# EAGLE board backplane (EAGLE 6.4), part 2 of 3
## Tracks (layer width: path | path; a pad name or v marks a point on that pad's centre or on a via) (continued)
HUB_!PWRON4  (via drill 0.6) (continued)
  Top 0.254: U1.23 113.83,195.54 113.03,196.34 97.79,196.34 97.28,195.83 21.34,195.83 v20.57,196.6 | S11.1 49.42,95.36 49.02,95.76 49.02,96.77 46.48,99.31 | v11.81,98.3 12.32,97.79 25.91,97.79 28.96,100.84 44.96,100.84 46.23,99.57 46.48,99.31 | v5.59,98.42 5.33,98.55 4.32,99.57 4.32,159 20.57,175.26 v20.57,188.85 | TP38.TESTPOINT 46.48,99.31
  Bottom 0.254: v20.57,196.6 v20.57,188.85 | v11.81,98.3 5.84,98.3 v5.59,98.42
HUB_!PWRON6  (via drill 0.6)
  Top 0.254: S12.1 153.3,67.17 v153.8,66.67 | U1.32 108.45,189.75 107.7,190.5 103.63,190.5 97.28,184.15 97.28,166.12 99.57,163.83 v99.57,161.42 | v99.57,157.1 100.08,156.59 100.08,100.08 100.84,99.31 103.76,99.31 v104.01,99.06 | v106.3,99.06 106.55,99.31 122.17,99.31 v122.56,98.93 | v126.11,98.93 v128.4,98.93 | v131.19,98.93 v134.75,98.93 | v137.54,98.93 138.3,98.93 140.97,96.27 140.97,90.68 v140.59,90.3 | v140.59,88.01 140.59,86.23 149.99,76.83 v149.99,74.93
  Bottom 0.254: v153.8,66.67 152.78,67.69 152.78,69.47 151.76,70.48 151.76,74.04 150.88,74.93 v149.99,74.93 | v99.57,161.42 v99.57,157.1 | v104.01,99.06 v106.3,99.06 | v122.56,98.93 v126.11,98.93 | v128.4,98.93 v131.19,98.93 | v134.75,98.93 v137.54,98.93 138.18,98.93 139.19,99.95 TP40.TESTPOINT | v140.59,90.3 v140.59,88.01
HUB_!PWRON7  (via drill 0.6)
  Top 0.254: S10.1 148.07,157.62 v146.18,159.51 | U1.36 111.04,187.75 110.74,187.45 110.74,186.69 103.38,179.32 103.38,173.23 111.76,165.1 117.35,165.1 | 117.35,165.1 118.36,165.1 | 118.36,165.1 123.19,165.1 v123.44,164.85 | v125.73,164.85 126.11,165.23 128.02,165.23 v128.4,164.85 | v130.68,164.85 130.94,165.1 134.49,165.1 v134.75,164.85 | v137.54,164.85 138.68,164.85 142.88,160.66 v142.88,160.15 | TP42.TESTPOINT 117.86,164.59 | 117.86,164.59 117.35,165.1 | 117.86,164.59 118.36,165.1
  Bottom 0.254: v123.44,164.85 v125.73,164.85 | v128.4,164.85 v130.68,164.85 | v134.75,164.85 v137.54,164.85 | v142.88,160.15 145.54,160.15 v146.18,159.51
HUB_CFG  (via drill 0.6)
  Top 0.254: U1.40 114.81,186.22 114.81,187.71 116.46,189.36 v116.84,189.36 | v123.32,183.39 123.44,183.51 126.36,183.51 127.51,184.66 TP28.TESTPOINT
  Bottom 0.254: v116.84,189.36 117.22,188.98 117.86,188.98 118.62,188.21 118.62,186.94 122.43,183.13 123.06,183.13 v123.32,183.39
HUB_DM1
  Top 0.254: R4.1 119.45,204.47 C6.1 119.45,203.28 119.13,202.95 119.13,197.89 arc-11 119,196.34 arc14 U1.13
HUB_DM2
  Top 0.254: U1.17 116.83,198.64 113.54,201.93 113.54,202.95 113.87,203.28 C4.1 113.79,203.78 R2.1
HUB_DM3
  Top 0.254: U1.21 114.83,196.07 108.03,202.87 C8.1 108.03,204.47 R6.1
HUB_DM4
  Top 0.254: U1.26 111.12,192.75 arc-9 109.75,192.86 arc8 108.38,192.99 C12.1 107.04,192.99 R10.1
HUB_DM6
  Top 0.254: U1.34 110.26,188.75 109.22,187.71 106.5,187.71 C14.1 105.66,187.78 R12.1
HUB_DM7
  Top 0.254: U1.38 113.83,185.46 106.61,178.23 C10.1 106.61,176.53 R8.1
HUB_DP1
  Top 0.254: R3.1 118.29,204.47 C5.1 118.29,203.28 118.62,202.95 118.62,197.89 arc-9 118.49,196.34 arc9 U1.14 118.34,194.81
HUB_DP2
  Top 0.254: U1.18 116.33,198.38 113.03,201.68 113.03,202.95 112.7,203.28 C3.1 112.78,203.78 R1.1
HUB_DP3
  Top 0.254: U1.22 114.33,195.81 106.86,203.28 C7.1 106.86,204.47 R5.1
HUB_DP4
  Top 0.254: U1.27 111.12,192.25 arc2 109.73,192.23 arc-2 108.41,192.2 C11.1 107.04,192.2 R9.1
HUB_DP6
  Top 0.254: U1.35 110.53,188.25 109.22,186.94 106.5,186.94 C13.1 106.35,186.94 R11.1
HUB_DP7
  Top 0.254: U1.39 114.33,185.19 107.52,178.38 C9.1 107.52,176.53 R7.1
HUB_PORTDIS  (via drill 0.6)
  Top 0.254: U1.42 115.83,186.69 v116.59,187.45 | v125.09,181.74 126.36,181.74 127,181.1 128.02,181.1 129.29,182.37 TP30.TESTPOINT
  Bottom 0.254: v116.59,187.45 122.05,181.74 v125.09,181.74
HUB_PORTPWR  (via drill 0.6)
  Top 0.254: U1.41 115.33,187.46 116.33,188.47 117.09,188.47 v117.73,187.96 | v124.21,182.63 127.25,182.63 TP29.TESTPOINT
  Bottom 0.254: v117.73,187.96 117.73,187.07 122.17,182.37 123.95,182.37 v124.21,182.63
MOD0_5V
  Top 0.254: 107.19,321.31 107.44,321.56 | S1.1 107.69,320.81 107.19,321.31 | C33.1 106.68,320.8 107.19,321.31
  Top 1.27: J0.2 58.67,357.63 95,357.63 107.44,345.44 107.44,321.56
MOD0_5V_METERED  (via drill 1.2)
  Top 0.254: 107.19,317.76 106.93,317.5 C88.1 | S13.3 96.59,312.12 96.52,312.05 96.34,312.24 | S13.2 95.94,312.63 96.34,312.24 | C76.1 96.01,311.91 96.34,312.24 | S1.3 107.19,317.5 106.93,317.25
  Top 1.27: v45.47,186.18 39.37,192.28 17.02,192.28 8.38,200.91 8.38,274.32 23.88,289.56 84.84,289.56 v91.95,296.67 | 96.52,306.32 96.52,312.05 | 96.52,306.32 106.93,316.74 106.93,317.25 106.93,317.5 | v91.95,301.75 96.52,306.32
  Bottom 0.508: v45.47,186.18 53.59,194.06 TP16.TESTPOINT
  Bottom 1.27: J4.7 50.01,181.63 v45.47,186.18 | v91.95,296.67 v91.95,301.75
MOD0_D+_HUB-SW
  Top 0.254: R1.2 112.78,205.99 113.03,206.25 113.03,357.38 114.55,358.9 114.55,360.17 113.75,360.98 D1.4 111.8,360.98 111.63,360.81 109.98,360.81 | 109.98,360.81 109.35,360.81 108.86,361.3 U20.3 | R50.2 110.49,360.3 109.98,360.81
MOD0_D-_HUB-SW
  Top 0.254: U20.5 108.86,362.1 109.35,362.58 110.24,362.58 | R2.2 113.79,205.99 113.54,206.25 113.54,357.12 115.06,358.65 115.06,361.19 113.97,362.27 D1.2 111.94,362.27 111.63,362.58 110.24,362.58 | R51.2 110.49,362.84 110.24,362.58
MOD0_IN
  Top 0.254: J0.10 69.59,336.55 U8.7
MOD0_ISO_I2C  (via drill 0.6)
  Top 0.254: U2.5 96.27,352.04 | 96.27,352.04 R63.2 | 96.27,352.04 99.31,352.04 106.43,344.93 106.43,322.71 v106.05,322.33 | v109.35,322.33 109.35,321.18 110.49,320.04 110.49,312.17 v109.98,311.66 | v107.7,311.66 107.7,305.31 106.93,304.55 U26.11 106.93,299.72 106.43,299.21 76.2,299.21 73.91,301.5 73.91,309.37 | 73.91,309.37 73.91,309.63 74.93,310.64 R1002.2 | TP1002.TESTPOINT 88.65,309.63 74.17,309.63 73.91,309.37
  Bottom 0.254: v106.05,322.33 v109.35,322.33 | v109.98,311.66 v107.7,311.66
MOD0_ISO_POWER
  Top 0.254: S1.4 107.69,318.27 107.95,318.01 107.95,316.48 109.11,315.33 R62.2 109.11,312.94 108.58,312.42 108.58,311.02 108.2,310.64 U26.10 108.2,299.97 106.93,298.7 75.95,298.7 73.41,301.24 73.41,313.44 73.66,313.69 | 73.66,313.69 74.68,314.71 R1001.2 | TP1001.TESTPOINT 88.65,313.69 73.66,313.69
MOD0_ISO_USB  (via drill 0.6)
  Top 0.203: U20.8 106.03,362.1 105.92,362.2 v105.92,362.97
  Top 0.254: v105.92,357.63 105.92,348.49 108.46,345.95 108.46,321.31 109.98,319.79 109.98,312.93 109.09,312.04 v109.09,310.13 | 102.11,304.29 102.73,304.91 S7.6 103.74,304.91 104.14,305.31 104.14,308.36 105.92,310.13 v106.81,310.13 | 102.11,304.29 R64.2 | 102.11,304.29 102.87,303.53 104.65,303.53 105.66,302.51 U26.12 105.66,300.23 105.16,299.72 76.45,299.72 74.42,301.75 74.42,305.31 | 74.42,305.31 74.42,306.07 74.93,306.58 R1003.2 | TP1003.TESTPOINT 88.65,305.56 74.68,305.56 74.42,305.31
  Bottom 0.254: v105.92,362.97 v105.92,357.63 | v109.09,310.13 v106.81,310.13
MOD0_OUT
  Top 0.254: J0.8 46.23,362.46 46.23,361.44 64.26,343.41 U14.7
MOD0_PPS
  Top 0.254: J0.7 44.96,363.78 44.96,361.95 69.85,337.05 U8.6
MOD0_SCL
  Top 0.203: 95.11,350.92 95.36,350.67 U2.6
  Top 0.254: J0.5 48.79,365.02 50.04,363.78 50.04,359.16 58.42,350.77 91.55,350.77 R34.2 95.11,350.92
MOD0_SDA
  Top 0.203: R33.2 95.14,350.15 95.25,350.27 U2.7
  Top 0.254: J0.6 48.77,362.46 48.77,359.66 58.15,350.28 93.73,350.27 93.84,350.15 R33.2
MOD0_USB+
  Top 0.254: J0.11 41.12,365.99 43.94,368.81 74.17,368.81 81.79,361.44 100.08,361.44 102.87,358.65 105.66,358.65 107.24,360.23 U20.1
MOD0_USB-
  Top 0.254: J0.12 39.88,363.73 39.88,365.51 43.69,369.32 74.42,369.32 82.04,361.95 100.08,361.95 103.12,365 105.66,365 107.24,363.42 U20.7
MOD0_USB_!EN  (via drill 0.6)
  Top 0.254: S13.4 97.24,312.97 v99.19,311.02 | S7.4 102.73,306.21 102.36,306.58 102.36,307.85 v101.22,308.99
  Bottom 0.254: v99.19,311.02 v101.22,308.99
MOD0_USB_VBUS
  Top 0.254: C77.1 91.95,325.88 93.22,324.61 | S13.7 95.94,319.71 96.14,319.91 | 96.14,319.91 96.27,320.04 | S13.6 96.59,319.46 96.14,319.91
  Top 0.762: C95.1 95.25,322.58
  Top 1.27: J0.13 38.58,364.97 36.83,363.22 36.83,361.7 73.66,324.87 92.99,324.87 92.99,324.84 93.22,324.61 95.25,322.58 96.27,321.56 96.27,320.04
MOD0_VCCIO  (via drill 1.2)
  Top 0.203: U2.8 95.36,349.87 95.25,349.76 95.25,349.25
  Top 0.254: v89.66,349 91.19,349 91.69,349.5 R34.1 92.46,348.85 R33.1 94.85,348.85 95.25,349.25 96.01,348.49 C22.1 | C52.1 94.74,342.65 | 94.74,342.65 94.74,342.89 U14.8 | C40.1 94.74,335.79 | 94.74,335.79 94.74,336.03 U8.8 | v89.66,335.28 94.23,335.28 94.74,335.79 | v89.66,342.14 94.23,342.14 94.74,342.65
  Top 1.27: J0.4 51.28,359.44 58.67,352.04 v89.66,352.04 | v89.66,349 v89.66,345.19 | v89.66,342.14 v89.66,338.84
  Bottom 1.27: v89.66,352.04 v89.66,349 | v89.66,345.19 v89.66,342.14 | v89.66,338.84 v89.66,335.28
MOD1_5V
  Top 0.254: C34.1 163.43,332.49 163.43,331.72 163.18,331.47 S2.1
  Top 1.27: J1.2 215.42,360.2 187.2,331.72 163.43,331.72
MOD1_5V_METERED  (via drill 1.2)
  Top 0.254: S14.2 149.31,357.7 C78.1 149.53,357.05 S14.3 | 155.82,331.72 156.18,331.36 C89.1 157.33,331.97 S2.3
  Top 1.27: v145.29,363.22 145.29,358.9 | 145.29,358.9 146.81,357.38 148.99,357.38 C78.1 | 145.29,358.9 145.29,339.09 152.66,331.72 155.82,331.72 | v28.7,190.25 16.51,190.25 6.6,200.15 6.6,274.83 12.45,280.67 12.45,294.39 6.6,300.23 6.6,340.87 39.88,374.14 77.72,374.14 83.57,368.3 96.77,368.3 102.87,374.4 137.16,374.4 v145.29,366.27
  Bottom 0.508: 30.48,188.47 30.73,188.47 33.02,190.75 49.02,190.75 53.59,195.33 59.69,195.33 TP17.TESTPOINT
  Bottom 1.27: J4.8 50.01,168.63 46.48,165.1 32.51,165.35 30.48,167.39 30.48,188.47 v28.7,190.25 | v145.29,366.27 v145.29,363.22
MOD1_D+_HUB-SW
  Top 0.203: U21.3 122.79,362.6
  Top 0.254: 122.79,362.6 122.17,363.22 120.9,363.22 | R3.2 118.36,205.99 118.62,206.25 118.62,356.62 116.84,358.39 116.84,361.7 118.07,362.93 D1.8 120.1,362.93 120.4,363.22 120.9,363.22 | R52.2 121.41,363.73 120.9,363.22
MOD1_D-_HUB-SW
  Top 0.203: U21.5 122.79,361.8
  Top 0.254: R4.2 119.38,205.99 119.13,206.25 119.13,356.87 117.35,358.65 117.35,360.93 118.04,361.62 D1.6 119.96,361.62 120.27,361.31 120.9,361.31 | 120.9,361.31 122.3,361.31 122.79,361.8 | R53.2 121.41,360.81 120.9,361.31
MOD1_IN
  Top 0.254: J1.10 205.26,360.96 195.83,351.53 U9.7
MOD1_ISO_I2C  (via drill 0.6)
  Top 0.254: U3.5 R66.2 158.13,336.95 157.73,336.55 157.23,336.55 155.45,334.77 v155.45,333.25 | v158.24,323.34 U27.11 v158.24,319.28 | v158.24,325.88 158.24,326.39 v155.45,329.18 | LED1005.A TP1005.TESTPOINT 161.29,310.64 158.24,313.69 v158.24,314.71
  Bottom 0.254: v155.45,329.18 v155.45,333.25 | v158.24,323.34 v158.24,325.88 | v158.24,314.71 v158.24,319.28
MOD1_ISO_POWER  (via drill 0.6)
  Top 0.254: v159.51,323.34 U27.10 v159.51,319.28 | S2.4 158.5,331.47 158.24,331.22 158.24,329.44 158.61,329.07 | R65.2 158.61,329.07 | LED1004.A TP1004.TESTPOINT v159.51,314.71 | v159.51,325.88 159.51,328.17 158.61,329.07
  Bottom 0.254: v159.51,323.34 v159.51,325.88 | v159.51,314.71 v159.51,319.28
MOD1_ISO_USB  (via drill 0.6)
  Top 0.203: U21.8 126.13,361.8 126.24,361.7 126.26,361.42
  Top 0.254: v156.97,323.34 U27.12 v156.97,319.28 | v156.97,325.88 144.27,338.58 144.27,350.5 v143.89,350.89 143.89,350.9 142.88,351.92 130.44,351.9 126.49,355.85 126.49,356.25 R67.2 126.49,356.98 v126.49,358.52 | 126.26,361.42 126.26,360.66 v126.49,360.43 | S8.6 148.48,349.87 147.46,350.89 v146.69,350.89 | LED1006.A TP1006.TESTPOINT 162.56,306.58 156.97,312.17 v156.97,314.71
  Bottom 0.254: v143.89,350.89 v146.69,350.89 | v156.97,323.34 v156.97,325.88 | v126.49,360.43 v126.49,358.52 | v156.97,314.71 v156.97,319.28
MOD1_OUT
  Top 0.254: J1.8 207.77,362.46 207.77,360.93 192.53,345.69 U15.7
MOD1_PPS
  Top 0.254: J1.7 206.5,363.73 206.5,361.44 196.09,351.03 U9.6
MOD1_SCL
  Top 0.203: U3.6 159.91,338.18 160.13,337.96 163.29,337.96
  Top 0.254: J1.5 210.34,364.97 211.58,363.73 211.58,361.95 187.56,337.93 R36.2 163.32,337.93 163.29,337.96
MOD1_SDA
  Top 0.203: U3.7 161.02,338.58
  Top 0.254: J1.6 210.34,361.47 187.45,338.58 161.02,338.58 161.04,338.57 R35.2
MOD1_USB+
  Top 0.254: J1.11 202.72,365.74 199.39,369.06 182.63,369.06 178.56,365 126.24,365 124.91,363.67 U21.1
MOD1_USB-
  Top 0.254: J1.12 202.67,362.48 201.42,363.73 201.42,366.27 199.14,368.55 182.88,368.55 178.82,364.49 132.84,364.49 128.27,359.41 126.24,359.41 124.91,360.73 U21.7
MOD1_USB_!EN  (via drill 0.6)
  Top 0.254: S8.4 148.7,351.93 v148.34,352.3 | v148.34,355.09 149.65,356.4 S14.4
  Bottom 0.254: v148.34,352.3 v148.34,355.09
MOD1_USB_VBUS
  Top 0.254: S14.7 156.39,357.7 156.59,357.5 | 156.59,357.5 156.72,357.38 | S14.6 156.14,357.05 156.59,357.5 | C79.1 163.83,357.38
  Top 0.762: C96.1 159.77,357.38
  Top 1.27: J1.13 193.06,365.02 185.42,357.38 163.83,357.38 159.77,357.38 156.72,357.38
MOD1_VCCIO  (via drill 1.2)
  Top 0.203: U3.8 159.91,338.98 160.02,339.09
  Top 0.254: U9.8 162.04,352.03 162.94,352.93 | 163.32,353.31 162.94,352.93 | C42.1 162.45,353.43 162.94,352.93 | U15.8 162.04,346.19 162.31,346.46 162.31,347.22 | 162.31,347.22 162.56,347.47 | C54.1 161.94,347.58 162.31,347.22 | 160.02,339.09 160.02,339.34 160.54,339.87 | v165.35,340.11 164.34,340.11 163.83,339.6 R36.1 162.93,339.23 162.29,339.87 R35.1 160.54,339.87 | 160.54,339.87 160.51,339.87 160.27,340.11 C24.1
  Top 1.27: J1.4 212.88,361.47 187.71,336.55 v165.35,336.55 | v165.35,347.47 162.56,347.47 | v165.35,353.31 163.32,353.31
  Bottom 1.27: v165.35,336.55 v165.35,340.11 v165.35,347.47 v165.35,353.31
MOD2_5V
  Top 0.254: C35.1 93.73,270.26 | 94.48,270.51 94.23,270.26 93.98,270.51 S3.1
  Top 1.27: 94.23,270.26 93.73,270.26 92.71,270.26 90.93,271.78 90.17,272.54 62.99,272.54 56.06,265.61 J2.2
MOD2_5V_METERED
  Top 0.254: S15.3 54.79,284.04 54.99,283.85 | 54.99,283.85 55.12,283.72 | S15.2 54.54,283.39 54.99,283.85 | C80.1 55.88,284.99 | C90.1 94.23,275.08 | 94.23,274.57 94.48,274.32 S3.3
  Top 0.508: 50.8,186.69 51.05,186.69 54.1,189.74 TP18.TESTPOINT
  Top 1.27: J4.9 47.47,181.33 50.8,184.66 50.8,186.69 43.18,194.31 17.53,194.31 10.16,201.68 10.16,273.56 24.38,287.78 53.85,287.78 | 53.85,287.78 81.79,287.78 94.23,275.34 94.23,275.08 94.23,274.57 | 53.85,287.78 55.88,285.75 55.88,284.99 55.88,284.48 55.12,283.72
MOD2_D+_HUB-SW
  Top 0.203: U22.3 95.65,228.33 95.76,228.22
  Top 0.254: R5.2 106.93,205.99 107.19,206.25 107.19,221.74 105.66,223.27 105.41,223.52 | 105.41,223.52 100.8,228.13 D2.8 98.85,228.13 98.81,228.09 arc-85 95.76,228.22 | R54.2 105.41,223.52
MOD2_D-_HUB-SW
  Top 0.203: U22.5 95.65,229.13 95.76,229.24
  Top 0.254: R6.2 107.95,205.99 107.7,206.25 107.7,222.76 107.44,223.01 106.93,223.52 | 106.93,223.52 101.02,229.43 D2.6 98.86,229.43 98.81,229.49 arc80 95.76,229.24 | R55.2 106.93,223.52
MOD2_IN
  Top 0.254: J2.10 43.66,262.41 67.06,239.01 U10.7
MOD2_ISO_I2C  (via drill 0.6)
  Top 0.254: U4.5 102.62,262.02 R69.2 102.87,262.75 102.87,268.48 | U28.11 99.57,273.81 102.87,270.51 102.87,268.48 | R1008.2 75.8,263.79 76.45,263.14 88.65,263.14 TP1008.TESTPOINT 97.03,264.16 99.82,266.95 v99.82,267.72 | v101.85,267.72 102.11,267.72 102.87,268.48
  Bottom 0.254: v99.82,267.72 v101.85,267.72
MOD2_ISO_POWER  (via drill 0.6)
  Top 0.254: 98.69,271.78 R68.2 | U28.10 98.3,272.8 | 98.3,272.8 98.81,272.29 R68.2 | S3.4 92.75,273.27 v92.71,273.3 | v97.28,273.3 97.79,273.3 98.3,272.8 | R1007.2 75.8,267.86 76.45,267.21 88.65,267.21 TP1007.TESTPOINT 94.74,268.22 95.76,267.21 96.77,267.21 97.54,267.97 97.54,271.02 98.19,271.67 R68.2
  Bottom 0.254: v92.71,273.3 v97.28,273.3
MOD2_ISO_USB  (via drill 0.6)
  Top 0.203: U22.8 92.69,229.13 92.46,229.36 92.46,229.87 v92.71,230.12
  Top 0.254: v92.71,232.41 92.71,234.44 v89.41,237.74 | U28.12 v100.84,274.07 | v96.77,275.84 95.76,275.84 v88.14,283.46 | v83.82,283.46 62.74,283.46 62.04,284.16 S9.6 | v89.41,241.05 v89.41,247.65 | v89.41,250.7 v89.41,254.51 | 96.52,262.89 v92.2,258.83 90.93,260.1 TP1009.TESTPOINT 88.65,259.08 76.45,259.08 75.8,259.73 R1009.2 | 96.52,262.89 100.84,267.21 v100.84,271.27 | R70.2 96.52,262.89
  Bottom 0.254: v92.71,230.12 v92.71,232.41 | v96.77,275.84 98.55,274.07 v100.84,274.07 v100.84,271.27 | v88.14,283.46 v83.82,283.46 | v89.41,237.74 v89.41,241.05 | v89.41,247.65 v89.41,250.7 | v89.41,254.51 89.41,257.56 90.68,258.83 v92.2,258.83
MOD2_OUT
  Top 0.254: J2.8 46.2,261.39 58.42,249.17 U16.7
MOD2_PPS
  Top 0.254: J2.7 46.15,268.15 44.96,266.95 44.96,261.87 67.31,239.52 U10.6
MOD2_SCL
  Top 0.203: U4.6 101.71,259.99 101.46,260.24
  Top 0.254: J2.5 48.74,267.49 50.04,266.19 50.04,265.18 59.18,256.03 92.2,256.03 96.27,260.1 99.31,260.1 99.46,260.24 R38.2 101.46,260.24
MOD2_SDA
  Top 0.203: 101.35,259.59 U4.7
  Top 0.254: J2.6 49,265.45 58.93,255.52 92.46,255.52 96.52,259.59 97.03,259.59 | 97.03,259.59 101.35,259.59 | R37.2 97.03,259.59
MOD2_USB+
  Top 0.203: U22.1 94.03,227.64 93.78,227.38
  Top 0.254: J2.11 41.07,268.15 39.88,266.95 39.88,264.67 75.95,228.6 86.87,228.6 88.9,226.57 92.96,226.57 93.78,227.38
MOD2_USB-
  Top 0.203: U22.7 94.03,230.07 93.98,230.12 93.78,230.32
  Top 0.254: J2.12 41.12,264.19 76.2,229.11 86.87,229.11 88.9,231.14 92.96,231.14 93.78,230.32
MOD2_USB_!EN  (via drill 0.6)
  Top 0.254: S15.4 53.54,285.69 v53.59,285.75 | 59.18,286.26 v58.93,286.26 59.44,286.26 59.55,286.15 S9.4
  Bottom 0.254: v53.59,285.75 54.1,286.26 v58.93,286.26
MOD2_USB_VBUS
  Top 0.254: C81.1 38.84,281.69 38.58,281.43 | C97.1 37.8,282.45 38.58,281.66 | S15.6 48.33,284.04 48.13,283.85 | 48.13,283.85 48.01,283.72 | S15.7 48.59,283.39 48.13,283.85
  Top 1.27: J2.13 38.58,281.43 38.58,281.66 40.64,283.72 48.01,283.72
MOD2_VCCIO  (via drill 1.2)
  Top 0.203: U4.8 101.71,259.19 101.35,258.83
  Top 0.254: 100.85,238.52 U10.8 100.6,238.52 100.33,238.25 100.33,237.74 C44.1 | U16.8 100.6,248.68 100.08,248.16 100.08,247.65 100.33,247.4 C56.1 | 98.55,257.92 R37.1 95.62,257.92 91.69,254 v91.19,254 | 98.55,257.92 R38.1 | 101.35,258.83 C26.1 99.03,257.44 98.55,257.92
  Top 1.27: v91.19,241.3 v91.19,247.4 91.19,247.65 100.08,247.65 | v91.19,237.74 100.33,237.74 | v91.19,257.3 59.69,257.3 51.38,265.61 J2.4 | v91.19,254 v91.19,250.95
  Bottom 1.27: v91.19,250.95 v91.19,247.4 | v91.19,241.3 v91.19,237.74 | v91.19,257.3 v91.19,254
MOD5_5V
  Top 0.254: C36.1 158.24,128.27 | 157.99,128.27 156.97,128.27 156.46,128.78 S4.1
  Top 1.27: J5.2 215.42,167.41 176.28,128.27 158.24,128.27 157.99,128.27
MOD5_5V_METERED  (via drill 1.2)
  Top 0.254: S16.3 147.39,161.47 147.19,161.67 | S16.2 147.65,162.12 147.19,161.67 | 147.19,161.67 147.07,161.8 | C82.1 146.81,161.8 | C91.1 152.54,129.79 152.15,129.79 152.66,129.28 S4.3
  Top 0.508: 49.3,166.9 50.57,166.9 51.31,167.64 51.31,179.07 53.59,181.36 60.71,181.36 62.48,183.13 62.48,186.44 TP19.TESTPOINT
  Top 1.27: 47.47,168.68 J4.10 49.3,166.9 57.71,158.5 v93.73,158.5 | v106.68,157.99 107.19,158.5 143.26,158.5 | 143.26,158.5 146.56,161.8 146.81,161.8 147.07,161.8 | 152.15,129.79 151.13,129.79 147.83,133.1 147.83,155.45 144.53,158.5 143.26,158.5 | v103.63,157.99 103.12,158.5 v96.77,158.5
  Bottom 1.27: v93.73,158.5 v96.77,158.5 | v103.63,157.99 v106.68,157.99
MOD5_D+_HUB-SW
  Top 0.203: U23.3 153.78,175.15
  Top 0.254: R7.2 107.44,175.01 111,171.45 137.67,171.45 arc27 138.68,171.7 arc-50 141.48,171.83 141.53,171.78 D3.2 144.34,171.78 147.72,175.15 148.84,175.15 | R56.2 149.24,175.55 148.84,175.15 | 153.78,175.15 153.65,175.16 arc84 151.13,175.39 arc-35 149.86,175.13 148.84,175.15
MOD5_D-_HUB-SW
  Top 0.203: U23.5 153.88,174.35
  Top 0.254: R8.2 106.68,175.01 110.74,170.94 137.67,170.94 arc-32 138.68,170.69 arc50 141.48,170.43 141.52,170.47 D3.4 143.81,170.47 147.68,174.35 150.11,174.35 arc-33 151.33,174.01 | R57.2 150.88,173.59 151.33,174.01 | 151.33,174.01 arc34 152.96,173.94 arc13 153.87,174.35 153.88,174.35
MOD5_IN  (via drill 0.6)
  Top 0.254: J5.10 205.26,164.11 184.91,143.76 165.86,143.76 v165.35,144.27 | U11.7 162.05,143.76 v162.31,144.02
  Bottom 0.254: v162.31,144.02 162.56,143.76 164.85,143.76 v165.35,144.27
MOD5_ISO_I2C  (via drill 0.6)
  Top 0.254: v145.41,133.73 145.8,134.11 145.8,143 145.03,143.76 145.03,145.8 144.53,146.3 U29.11 | v149.22,134.37 R72.2 155.19,134.48 U5.5 | LED1011.A TP1011.TESTPOINT 156.46,116.84 144.27,129.03 v144.27,130.3
  Bottom 0.254: v149.22,134.37 148.59,133.73 v145.41,133.73 144.27,132.59 v144.27,130.3
MOD5_ISO_POWER  (via drill 0.6)
  Top 0.254: v145.41,132.46 144.53,133.35 144.53,134.11 145.29,134.87 145.29,142.75 144.53,143.51 144.53,144.78 144.27,145.03 U29.10 | v149.61,133.22 153.66,133.22 153.8,133.1 154.56,132.33 | 154.56,132.33 R71.2 | S4.4 153.8,128.78 v153.42,128.4 | v154.69,131.32 154.69,132.21 154.56,132.33 | LED1010.A TP1010.TESTPOINT 157.23,120.9 v153.42,124.71
  Bottom 0.254: v145.41,132.46 148.84,132.46 v149.61,133.22 | v154.69,131.32 154.69,129.79 153.42,128.52 v153.42,128.4 v153.42,124.71
MOD5_ISO_USB  (via drill 0.6)
  Top 0.203: U23.8 156.61,174.35 156.97,173.99
  Top 0.254: 156.97,173.99 v156.97,173.23 | v156.97,171.32 157.35,171.32 162.56,166.12 v162.56,163.96 | S10.6 156.46,157.62 | 156.46,157.62 R73.2 156.97,159 157.86,159.89 v162.56,159.89 | v149.22,150.88 149.22,151.51 151.64,153.92 154.94,153.92 155.96,154.94 155.96,157.11 156.46,157.62 | v146.43,150.88 145.29,149.73 145.29,148.34 144.53,147.57 U29.12 142.49,147.57 142.24,147.32 142.24,144.53 142.49,144.27 143.26,144.27 143.76,143.76 143.76,142.49 141.99,140.72 v141.99,138.18 | LED1012.A TP1012.TESTPOINT 159.77,112.78 141.99,130.56 v141.99,134.87
  Bottom 0.254: v156.97,173.23 v156.97,171.32 | v162.56,163.96 v162.56,159.89 | v146.43,150.88 v149.22,150.88 | v141.99,134.87 v141.99,138.18
MOD5_OUT  (via drill 0.6)
  Top 0.254: J5.8 207.7,168.73 206.5,169.93 204.72,169.93 203.96,169.16 203.96,163.58 191,150.62 v165.35,150.62 | U17.7 v162.3,150.62 v162.31,150.62
  Bottom 0.254: v162.31,150.62 v165.35,150.62
MOD5_PPS  (via drill 0.6)
  Top 0.254: J5.7 207.8,171.17 209.04,169.93 209.04,167.13 185.17,143.26 165.61,143.26 v165.35,143 | U11.6 161.8,143.26 v162.31,142.75
  Bottom 0.254: v162.31,142.75 162.81,143.26 165.1,143.26 v165.35,143
MOD5_SCL
  Top 0.203: 156.61,136 156.36,136.25 U5.6
  Top 0.254: J5.5 210.49,171.27 211.58,170.18 211.58,168.15 179.44,136 R40.2 156.61,136
MOD5_SDA
  Top 0.203: U5.7 160.16,136.65
  Top 0.254: J5.6 210.34,167.66 179.32,136.65 161.43,136.65 | 160.16,136.65 161.15,136.65 | 161.15,136.65 161.43,136.65 | 161.43,136.65 R39.2 161.15,136.65
MOD5_USB+
  Top 0.203: U23.1 155.39,175.97
  Top 0.254: 155.39,175.97 156.72,177.29 159.51,177.29 161.8,175.01 198.98,175.01 J5.11
MOD5_USB-
  Top 0.203: U23.7 155.39,173.54
  Top 0.254: 155.39,173.54 156.72,172.21 159.51,172.21 161.8,174.5 198.63,174.5 201.42,171.7 201.42,170.03 J5.12
MOD5_USB_!EN
  Top 0.254: S10.4 154.07,156.32 153.67,156.72 153.67,158.75 152.65,159.77 149.61,159.77 149.16,160.22 S16.4
MOD5_USB_VBUS
  Top 0.254: C83.1 160.53,161.8 | S16.7 154.62,162.12 154.81,161.93 | 154.81,161.93 154.94,161.8 | S16.6 154.36,161.47 154.81,161.93
  Top 0.762: C98.1 156.97,161.8
  Top 1.27: J5.13 192.35,171.27 182.88,161.8 160.53,161.8 156.97,161.8 154.94,161.8
MOD5_VCCIO  (via drill 1.2)
  Top 0.203: U5.8 156.1,137.05 156.34,137.29
  Top 0.254: 156.34,137.29 156.46,137.29 | 156.46,137.29 159.24,137.29 R40.1 159.91,137.3 160.53,137.92 161.4,137.92 R39.1 163.69,138.06 v163.83,137.92 | U11.8 157.21,144.26 157.23,144.27 | 157.23,144.27 157.73,144.78 C46.1 | 157.23,144.27 161.04,144.27 161.8,145.03 162.81,145.03 163.83,144.02 | 157.23,151.13 157.21,151.12 U17.8 156.76,151.13 157.48,151.13 158.5,151.89 | C58.1 158.5,151.89 | C28.1 157.23,138.05 156.46,137.29 | 158.35,152.15 158.35,152 158.5,151.89
  Top 1.27: J5.4 212.88,167.41 180.34,134.62 v163.83,134.62 | v163.83,137.92 163.83,144.02 163.83,151.13 162.81,152.15 158.35,152.15
  Bottom 1.27: v163.83,134.62 v163.83,137.92
MOD6_5V  (via drill 1.2)
  Top 0.254: 29.21,89.66 29.21,90.31 C37.1 29.46,90.68 28.7,91.44 S5.1
  Top 1.27: v36.32,86.87 32,86.87 29.21,89.66
  Bottom 1.27: J6.2 51.56,69.6 38.1,69.6 36.32,71.37 v36.32,86.87
MOD6_5V_METERED
  Top 0.254: C84.1 38.61,99.82 38.73,99.69 | S17.2 38.93,99.5 38.73,99.69 | S17.3 38.28,99.24 38.73,99.69 | 28.96,96.77 28.7,96.52 29.46,95.76 C92.1 29.21,95.39 S5.3
  Top 0.508: J4.11 44.93,171.22 46.1,170.05 48.26,170.05 48.77,170.56 48.77,180.34 52.07,183.64 TP20.TESTPOINT
  Top 1.27: J4.11 44.93,173.51 41.66,176.78 25.91,176.78 7.11,157.99 7.11,101.09 11.43,96.77 28.96,96.77 29.72,97.54 34.04,97.54 36.32,99.82 38.61,99.82
MOD6_D+_HUB-SW
  Top 0.203: U24.3 96.75,88.12
  Top 0.254: R9.2 98.68,192.15 94.74,188.21 94.74,164.59 95.5,163.83 95.5,101.85 | 95.5,101.85 95.5,99.57 102.87,92.2 102.87,88.9 101.89,87.92 D4.8 99.86,87.92 99.82,87.88 arc-60 96.77,88.11 96.75,88.12 | R58.2 96.27,102.62 95.5,101.85
MOD6_D-_HUB-SW
  Top 0.203: U24.5 96.82,88.92
  Top 0.254: R10.2 98.81,193.04 94.23,188.47 94.23,164.34 95,163.58 95,101.85 | 95,101.85 95,99.31 102.36,91.95 102.36,89.92 101.67,89.22 D4.6 99.88,89.22 99.69,89.28 arc60 96.83,88.92 96.82,88.92 | R59.2 94.23,102.62 95,101.85
MOD6_IN
  Top 0.254: J6.10 43.66,66.57 62.23,48.01 U12.7
MOD6_ISO_I2C  (via drill 0.6)
  Top 0.254: U6.5 R75.2 97.17,64.88 96.52,65.53 96.52,69.6 97.28,70.36 | U30.11 v102.11,75.18 | v99.31,72.39 97.28,70.36 | R1014.2 75.8,69.74 76.45,69.09 88.39,69.09 TP1014.TESTPOINT 97.28,70.36
  Bottom 0.254: v102.11,75.18 v99.31,72.39
MOD6_ISO_POWER  (via drill 0.6)
  Top 0.254: 26.85,92.49 R74.2 | R74.2 26.81,90.54 31.75,85.6 34.8,85.6 37.08,83.31 37.08,71.63 38.1,70.61 38.86,70.61 65.79,43.43 103.89,43.43 104.14,43.69 105.16,43.69 v105.66,44.2 | v106.93,51.31 106.93,61.09 v107.7,61.85 | v107.7,64.14 107.7,75.18 106.43,76.45 U30.10 91.69,76.45 TP1013.TESTPOINT 88.39,73.15 76.45,73.15 75.8,73.8 R1013.2 | S5.4 27.65,93.94 26.81,93.11 R74.2
  Bottom 0.254: v106.93,51.31 106.43,50.8 106.43,44.96 v105.66,44.2 | v107.7,64.14 v107.7,61.85
MOD6_ISO_USB  (via drill 0.6)
  Top 0.203: U24.8 94.22,88.92 93.73,89.41 v93.73,89.66
  Top 0.254: v106.3,64.14 107.19,65.02 107.19,73.15 106.43,73.91 U30.12 94.74,73.91 v92.96,72.14 | v106.3,61.85 106.43,61.72 106.43,52.58 v105.92,52.07 | v104.65,42.8 104.52,42.93 65.02,42.93 36.58,71.37 36.58,83.06 34.54,85.09 30.48,85.09 24.26,91.31 v24.26,94.87 | v44.2,95.25 47.5,95.25 47.61,95.36 S11.6 48.07,94.93 48.51,94.49 52.72,94.49 | v93.73,91.69 93.22,91.19 89.15,91.19 85.85,94.49 52.72,94.49 | v27.69,98.3 28.32,98.93 v33.15,98.93 | 52.72,94.49 R76.2 | R1015.2 75.8,65.42 76.45,64.77 88.39,64.77 TP1015.TESTPOINT 92.2,68.58 v92.96,68.58
  Bottom 0.254: v93.73,89.66 v93.73,91.69 | v106.3,64.14 v106.3,61.85 | v105.92,52.07 105.92,45.72 104.65,44.45 v104.65,42.8 | v44.2,95.25 43.18,96.27 43.18,97.28 42.8,97.66 34.42,97.66 v33.15,98.93 | v24.26,94.87 v27.69,98.3 | v92.96,72.14 v92.96,68.58
MOD6_OUT
  Top 0.254: U18.7 56.13,55.63 46.2,65.56 J6.8
MOD6_PPS
  Top 0.254: J6.7 44.96,73.15 44.96,66.04 62.49,48.51 U12.6
MOD6_SCL
  Top 0.203: U6.6 96.63,63.65 96.52,63.75
  Top 0.254: J6.5 48.74,73.69 50.04,72.39 50.04,70.61 58.17,62.48 90.42,62.48 91.69,63.75 94.49,63.75 | 94.49,63.75 96.52,63.75 | R42.2 94.49,63.75
MOD6_SDA
  Top 0.203: U6.7 96.52,63.25
  Top 0.254: J6.6 48.74,71.14 57.91,61.98 90.68,61.98 91.95,63.25 92.2,63.25 | 92.2,63.25 96.52,63.25 | R41.2 92.2,63.25
MOD6_USB+
  Top 0.203: U24.1 95.3,87.43 94.23,86.36
  Top 0.254: 94.23,86.36 91.44,86.36 89.41,88.39 55.12,88.39 J6.11
MOD6_USB-
  Top 0.203: U24.7 95.3,89.61 94.23,90.68
  Top 0.254: 94.23,90.68 91.19,90.68 89.41,88.9 54.86,88.9 41.66,75.69 40.64,75.69 39.88,74.93 39.88,73.1 J6.12
MOD6_USB_!EN  (via drill 0.6)
  Top 0.254: S17.4 37.28,97.73 v36.32,96.77 | v42.16,96.77 42.16,97.54 42.93,98.3 46.74,98.3 47.24,97.79 47.24,97.03 47.61,96.66 S11.4
  Bottom 0.254: v36.32,96.77 v42.16,96.77
MOD6_USB_VBUS
  Top 0.254: 38.84,90.42 38.58,90.17 | C85.1 38.58,87.12 | S17.6 38.28,92.48 38.46,92.3 | 38.46,92.3 38.58,92.18 | S17.7 38.93,92.78 38.46,92.3
  Top 0.762: C99.1 38.84,90.42
  Top 1.27: J6.13 38.58,87.12 38.58,90.17 38.58,92.18
MOD6_VCCIO  (via drill 1.2)
  Top 0.203: U6.8 96.75,62.85 96.65,62.74
  Top 0.254: 96.65,62.74 96.52,62.61 C30.1 96.12,61.61 95.14,62.6 R42.1 93.84,62.6 92.95,61.71 R41.1 92.19,61.72 91.19,61.72 90.17,60.71 v89.66,60.71 | 94.63,46.74 C48.1 95.25,46.99 95.77,47.51 U12.8 | U18.8 95.77,55.13 95.25,54.61 95.25,54.36 | C60.1 95.25,54.36 | 94.74,54.36 95.25,54.36
  Top 1.27: J6.4 51.33,71.86 59.44,63.75 v89.66,63.75 | v89.66,60.71 v89.66,57.4 | v89.66,50.29 v89.66,54.36 94.74,54.36 | v89.66,46.74 94.63,46.74 94.74,46.74
  Bottom 1.27: v89.66,63.75 v89.66,60.71 | v89.66,57.4 v89.66,54.36 | v89.66,50.29 v89.66,46.74
MOD7_5V
  Top 0.254: 152.91,43.94 152.9,43.94 152.91,43.94 152.78,44.07 | C38.1 152.03,44.81 152.78,44.07 | S6.1 152.15,43.44 152.78,44.07
  Top 1.27: J7.2 215.42,71.14 188.21,43.94 152.91,43.94
MOD7_5V_METERED  (via drill 0.6, 1.2)
  Top 0.254: S18.2 149.42,71.95 149.1,71.63 149.42,71.3 S18.3 | C86.1 149.1,71.88 | 149.1,44.2 149.36,43.94 S6.3 | C93.1 148.84,43.94 149.1,44.2 | 149.1,44.7 149.1,44.45 149.1,44.2
  Top 0.508: v52.58,182.37 59.69,182.37 TP21.TESTPOINT
  Top 1.27: 149.1,71.88 149.1,71.63 v149.1,69.09 | v149.1,64.64 v149.1,58.29 | v149.1,55.5 v149.1,52.2 | v149.1,48.51 149.1,44.7 | 149.1,44.45 149.1,8.13 145.29,4.32 95.5,4.32 91.69,8.13 87.88,8.13 84.07,4.32 12.45,4.32 4.32,12.45 4.32,88.14 8.38,92.2 8.38,97.54 5.33,100.58 5.33,158.5 v32.26,185.42
  Bottom 0.508: J4.12 45.03,168.73 46.23,170.05 50.8,170.05 51.31,170.56 51.31,181.1 v52.58,182.37
  Bottom 1.27: v149.1,69.09 v149.1,64.64 | v149.1,58.29 v149.1,55.5 | v149.1,52.2 v149.1,48.51 | J4.12 44.93,168.63 43.18,166.88 33.78,166.88 32.26,168.4 v32.26,185.42
MOD7_D+_HUB-SW
  Top 0.203: 146.81,89.92 arc31 U25.3
  Top 0.254: R11.2 104.39,186.94 100.84,183.39 100.84,168.15 105.41,163.58 105.41,92.2 104.9,91.69 104.9,90.42 105.45,89.88 D4.4 107.4,89.88 107.44,89.92 arc-60 110.49,89.66 arc33 111.25,89.41 116.08,89.41 | 116.08,89.41 144.53,89.41 arc23 145.8,89.92 arc-45 146.81,89.92 | R60.2 116.84,90.17 116.08,89.41
MOD7_D-_HUB-SW
  Top 0.203: 146.94,88.52 arc-52 U25.5
  Top 0.254: R12.2 104.39,187.71 100.33,183.64 100.33,167.89 104.9,163.32 104.9,92.46 104.39,91.95 104.39,89.41 105.16,88.65 106.46,88.65 D4.2 106.6,88.65 107.44,88.65 arc60 110.24,88.65 arc-32 111.25,88.9 116.33,88.9 | 116.33,88.9 144.53,88.9 arc-44 145.8,88.52 arc87 146.94,88.52 | R61.2 116.84,88.39 116.33,88.9
MOD7_IN
  Top 0.254: J7.10 205.21,67.79 194.81,57.4 U13.7
MOD7_ISO_I2C  (via drill 0.6)
  Top 0.254: U7.5 155.19,49.02 | 155.19,49.02 155.19,47.86 R78.2 | 155.19,49.02 154.69,48.51 153.29,48.51 152.02,49.78 148.08,49.78 v147.7,49.4 | v147.57,51.69 147.7,51.82 147.7,55.88 v147.57,56.01 | v146.81,58.55 146.81,65.53 146.05,66.29 | 146.05,66.29 U31.11 | LED1017.A TP1017.TESTPOINT 157.48,70.1 155.96,68.58 155.96,67.56 154.18,65.79 152.91,65.79 152.15,66.55 146.3,66.55 146.05,66.29
  Bottom 0.254: v147.7,49.4 147.7,51.56 v147.57,51.69 | v147.57,56.01 146.81,56.77 v146.81,58.55
MOD7_ISO_POWER  (via drill 0.6)
  Top 0.254: v145.54,58.55 145.54,58.67 146.3,59.44 146.3,63.75 145.03,65.02 U31.10 142.24,65.02 141.73,65.53 141.73,75.44 142.49,76.2 146.18,76.2 v147.07,77.22 | v146.3,56.01 v146.3,51.69 | v146.3,49.4 146.3,46.61 v147.7,45.21 | 152.64,42.04 R77.2 152,42.05 151.76,42.29 v150.88,42.29 150.5,42.29 150.28,42.51 S6.4 | LED1016.A TP1016.TESTPOINT | v158.5,76.71 158.5,77.98 156.72,79.76 v152.53,79.76
  Bottom 0.254: v145.54,58.55 145.54,56.77 v146.3,56.01 | v146.3,51.69 v146.3,49.4 | v147.7,45.21 149.61,43.18 150.5,42.29 v150.88,42.29 | TP1016.TESTPOINT 160.78,74.42 v158.5,76.71 | v152.53,79.76 149.61,79.76 v147.07,77.22
MOD7_ISO_USB  (via drill 0.6)
  Top 0.203: 150.62,88.39 150.26,88.75 U25.8
  Top 0.254: v150.88,73.79 150.88,84.33 | 150.88,84.33 v150.88,86.23 | v150.88,88.01 150.62,88.39 | R79.2 151.13,84.07 150.88,84.33 | U31.12 144.27,67.56 144.67,67.17 S12.6 151.5,67.17 151.89,67.56 v151.89,69.09 | LED1018.A TP1018.TESTPOINT 163.32,66.04 160.02,69.34 157.48,69.34 156.46,68.33 156.46,67.31 155.19,66.04 v155.19,65.28
  Bottom 0.254: v150.88,86.23 v150.88,88.01 | v150.88,73.79 150.88,70.1 v151.89,69.09 151.89,67.06 153.67,65.28 v155.19,65.28
MOD7_OUT
  Top 0.254: J7.8 207.03,71.86 205.74,73.15 204.72,73.15 203.96,72.39 203.96,67.31 200.91,64.26 U19.7
MOD7_PPS
  Top 0.254: U13.6 195.08,56.9 209.04,70.87 209.04,73.15 J7.7
MOD7_SCL
  Top 0.203: U7.6 156.1,49.89 156.34,49.66
  Top 0.254: 210.31,74.42 J7.5 211.58,73.15 211.58,71.37 210.82,70.61 210.31,70.61 189.48,49.78 160.78,49.78 160.64,49.64 R44.2 160.51,49.66 156.34,49.66
MOD7_SDA
  Top 0.203: U7.7 156.21,50.29
  Top 0.254: J7.6 210.34,71.4 189.23,50.29 158.75,50.29 R43.2 158.64,50.29 156.21,50.29
MOD7_USB+
  Top 0.203: U25.1 149.04,90.37 149.86,91.19
  Top 0.254: 149.86,91.19 153.92,91.19 155.7,89.41 187.71,89.41 J7.11
MOD7_USB-
  Top 0.203: U25.7 149.04,87.94 149.86,87.12
  Top 0.254: 149.86,87.12 153.92,87.12 155.7,88.9 187.45,88.9 201.42,74.93 201.42,73.15 J7.12
MOD7_USB_!EN
  Top 0.254: S12.4 150.94,70.64 S18.4
MOD7_USB_VBUS
  Top 0.254: S18.6 156.14,71.3 156.34,71.5 | 156.34,71.5 156.46,71.63 | S18.7 155.88,71.95 156.34,71.5 | C87.1 164.34,77.47
  Top 0.762: C100.1 162.31,77.47
  Top 1.27: J7.13 200.13,74.4 200.13,74.45 197.1,77.47 164.34,77.47 162.31,77.47 156.46,71.63
MOD7_VCCIO  (via drill 1.2)
  Top 0.203: U7.8 156.1,50.69 156.46,51.05 | C32.1 156.46,52.32 156.84,51.94
  Top 0.254: U19.8 156.96,64.76 157.73,65.53 | C62.1 158.24,66.04 | C50.1 157.73,58.67 | U13.8 157.21,57.9 157.48,58.17 157.48,58.67 | 156.46,51.05 156.46,51.56 | R44.1 159.62,50.94 159,51.56 158.38,51.56 R43.1 157.59,51.7 157.1,52.2
  Top 1.27: J7.4 212.88,71.14 190.25,48.51 v162.56,48.51 | v160.53,62.48 v160.53,58.67 157.73,58.67 157.48,58.67 | v160.53,66.04 158.24,66.04 | 156.46,51.56 156.84,51.94 157.1,52.2 157.73,52.83 160.53,52.83 160.78,53.09 | v162.56,51.56 162.31,51.56 160.78,53.09 | 160.78,53.09 160.53,53.34 v160.53,55.63
  Top 1.422: 158.24,66.04 157.73,65.53
  Bottom 1.27: v162.56,48.51 v162.56,51.56 | v160.53,55.63 v160.53,58.67 | v160.53,62.48 v160.53,66.04
MOD_SCL  (via drill 0.6)
  Top 0.203: U3.3 157.99,338.58 | U5.3 154.18,136.65 153.92,136.4 153.67,136.4 | 153.92,50.29 U7.3 | 99.06,63.25 U6.3 | U4.3 103.89,259.59 | U2.3 100.33,350.27
  Top 0.254: v153.67,338.07 154.18,338.58 157.99,338.58 | v128.91,170.05 129.29,169.67 129.29,161.8 v128.91,161.42 | v128.91,157.1 128.91,156.84 129.29,156.46 129.29,136.78 | 129.29,136.78 129.29,90.55 v129.03,90.3 | v128.91,172.34 128.91,172.59 140.97,184.66 166.37,184.66 169.93,188.21 195.83,188.21 210.34,202.72 J3.24 210.34,209.78 209.04,211.07 209.04,212.85 207.77,214.12 193.8,214.12 149.1,258.83 v146.94,258.83 146.56,259.21 146.56,261.37 139.7,268.22 139.7,326.26 v140.21,326.77 147.19,333.76 v147.57,333.76 | 153.67,136.4 149.86,136.4 v149.22,135.64 | v143.89,135.64 143.38,136.14 137.54,136.14 v137.03,135.64 | v134.24,135.64 133.86,136.14 131.06,136.14 130.81,135.89 v130.68,135.89 | v128.4,135.89 129.29,136.78 | v129.03,88.01 129.03,87.88 129.54,87.38 129.54,81.92 v129.03,81.41 | v129.03,78.61 129.03,75.18 v129.41,74.8 | 153.92,50.29 139.7,50.29 131.32,58.67 131.32,72.9 v131.06,73.15 130.56,73.15 120.65,63.25 99.06,63.25 | 103.89,259.59 111.76,259.59 v112.14,259.97 | v114.43,259.97 114.81,259.59 117.35,259.59 v117.73,259.97 | v120.02,259.97 120.4,259.59 141.73,259.59 | 141.73,259.59 142.75,259.59 | 142.75,259.59 v145.03,259.59 | 100.33,350.27 105.92,344.68 105.92,326.9 v105.54,326.52 | v137.29,326.9 136.53,326.14 120.4,326.14 v120.02,326.52 | v117.73,326.52 117.35,326.14 114.81,326.14 v114.43,326.52 | v112.14,326.52 111.76,326.14 109.73,326.14 v109.35,326.52 | R49.1 142.24,260.1 | 142.24,260.1 141.73,259.59 | 142.24,260.1 142.75,259.59 | v143.76,256.16 143.76,255.52 TP6.TESTPOINT
  Bottom 0.203: 137.41,326.77 v137.29,326.9
  Bottom 0.254: v153.67,338.07 151.89,338.07 v147.57,333.76 | v128.91,172.34 v128.91,170.05 | v128.91,161.42 v128.91,157.1 | v149.22,135.64 v143.89,135.64 | v137.03,135.64 v134.24,135.64 | v130.68,135.89 v128.4,135.89 | v129.03,90.3 v129.03,88.01 | v129.03,81.41 v129.03,78.61 | v129.41,74.8 v131.06,73.15 | v112.14,259.97 v114.43,259.97 | v117.73,259.97 v120.02,259.97 | v140.21,326.77 137.41,326.77 | v120.02,326.52 119.63,326.14 118.11,326.14 v117.73,326.52 | v114.43,326.52 114.05,326.14 112.52,326.14 v112.14,326.52 | v109.35,326.52 108.97,326.14 105.92,326.14 v105.54,326.52 | v146.94,258.83 145.8,258.83 v145.03,259.59 143.76,258.32 v143.76,256.16
MOD_SDA  (via drill 0.6)
  Top 0.203: U3.2 158.1,338.98 157.99,339.09 | U5.2 154.07,137.05 153.92,136.91 153.67,136.91 | U7.2 154.03,50.69 153.92,50.8 | U6.2 98.95,62.85 99.06,62.74 | U4.2 103.52,259.19 103.63,259.08 | U2.2 99.97,349.87
  Top 0.254: v153.67,339.6 154.18,339.09 157.99,339.09 | 149.1,259.59 194.06,214.63 208.03,214.63 210.34,212.32 J3.23 210.34,211.3 211.58,210.06 211.58,203.2 196.09,187.71 170.18,187.71 166.62,184.15 141.22,184.15 130.18,173.1 v130.18,172.34 | 149.1,259.59 140.21,268.48 140.21,325.12 v140.72,325.63 v147.57,332.49 | v130.18,170.05 129.79,169.67 129.79,161.8 v130.18,161.42 | v130.18,157.1 130.18,156.84 129.79,156.46 129.79,137.92 | 129.79,137.92 129.79,90.81 v130.3,90.3 | 153.67,136.91 v149.22,136.91 | v143.89,136.91 143.64,136.65 137.41,136.65 137.16,136.91 v137.03,136.91 | v134.24,136.91 134.11,136.91 133.86,136.65 131.06,136.65 129.79,137.92 | v130.3,88.01 130.05,87.76 130.05,81.66 v130.3,81.41 | v130.3,78.61 v130.3,75.56 | v131.95,74.04 131.95,73.03 131.83,72.9 131.83,58.93 139.95,50.8 153.92,50.8 | v130.43,71.37 129.54,71.37 120.9,62.74 99.06,62.74 | 103.63,259.08 111.76,259.08 v112.14,258.7 | v114.43,258.7 114.81,259.08 117.35,259.08 v117.73,258.7 | v120.02,258.7 120.4,259.08 139.7,259.08 | 139.7,259.08 141.73,259.08 | 141.73,259.08 142.75,259.08 | 142.75,259.08 144.27,259.08 v145.03,258.32 | v137.29,325.63 120.4,325.63 v120.02,325.25 | v117.73,325.25 117.35,325.63 114.81,325.63 v114.43,325.25 | v112.14,325.25 111.76,325.63 109.73,325.63 v109.35,325.25 | v105.54,325.25 104.65,326.14 104.65,326.9 105.41,327.66 105.41,344.42 99.97,349.87 | 149.1,259.59 147.96,259.59 v147.83,259.71 | R48.1 142.24,258.57 | 142.24,258.57 141.73,259.08 | 142.24,258.57 142.75,259.08 | TP5.TESTPOINT 137.16,256.54 139.7,259.08
  Bottom 0.254: v153.67,339.6 152.65,338.58 151.64,338.58 147.83,334.77 147.32,334.77 146.56,334.01 146.56,333.5 v147.57,332.49 | v130.18,172.34 v130.18,170.05 | v130.18,161.42 v130.18,157.1 | v149.22,136.91 v143.89,136.91 | v137.03,136.91 v134.24,136.91 | v130.3,90.3 v130.3,88.01 | v130.3,81.41 v130.3,78.61 | v130.3,75.56 130.43,75.56 v131.95,74.04 131.95,73.03 131.83,72.9 131.83,71.88 131.32,71.37 v130.43,71.37 | v112.14,258.7 v114.43,258.7 | v117.73,258.7 v120.02,258.7 | v140.72,325.63 v137.29,325.63 | v120.02,325.25 119.63,325.63 118.11,325.63 v117.73,325.25 | v114.43,325.25 114.05,325.63 112.52,325.63 v112.14,325.25 | v109.35,325.25 108.97,325.63 105.92,325.63 v105.54,325.25 | v147.83,259.71 147.83,258.57 147.19,257.94 145.41,257.94 v145.03,258.32
N$1
  Top 0.406: R1001.1 LED1001.A
N$2
  Top 0.406: R1002.1 LED1002.A
N$3
  Top 0.406: R1003.1 LED1003.A
N$4
  Top 0.254: LED1007.A R1007.1
N$5
  Top 0.254: LED1008.A R1008.1
N$6
  Top 0.254: LED1009.A R1009.1
N$7
  Top 0.254: LED1013.A R1013.1
N$8
  Top 0.254: LED1014.A R1014.1
N$9
  Top 0.254: LED1015.A R1015.1
N$10
  Top 0.254: LED1004.C R1004.2
N$11
  Top 0.254: LED1005.C R1005.2
N$12
  Top 0.254: U1.2 121.74,188.25 R25.2
N$13
  Top 0.254: LED1006.C R1006.2
N$14
  Top 0.254: R26.1 116.84,182.12 | 116.84,182.12 116.84,176.78 116.33,176.28 Y1.1 | C2.2 116.59,181.86 116.84,182.12
N$15
  Top 0.254: R1010.2 LED1010.C
N$16
  Top 0.254: R1011.2 LED1011.C
N$17
  Top 0.203: U20.2 107.64,357.04
  Top 0.254: 107.64,357.04 R13.1
N$18
  Top 0.203: U25.6 148.64,86.78 R24.1
N$19
  Top 0.203: U25.2 148.64,91.53 R23.1
N$20
  Top 0.203: U24.6 95.7,89.61 96.01,89.92
  Top 0.254: 96.01,89.92 R22.1
N$21
  Top 0.203: U24.2 95.7,87.18 96.01,86.87
  Top 0.254: 96.01,86.87 R21.1
N$22
  Top 0.203: U23.6 154.99,173.54 154.69,173.23
  Top 0.254: 154.69,173.23 R20.1
N$23
  Top 0.203: U23.2 154.99,175.97 154.69,176.28
  Top 0.254: R19.1 154.18,176.78 154.69,176.28
N$24
  Top 0.203: 95.25,226.82 94.43,227.64 U22.2
  Top 0.254: R17.1 95.25,226.82
N$25
  Top 0.203: 95.25,230.89 94.43,230.07 U22.6
  Top 0.254: R18.1 95.25,230.89
N$26
  Top 0.203: U21.6 124.51,360.59
  Top 0.254: 124.51,360.59 124.51,357.07 R16.1
N$27
  Top 0.203: U21.2 124.51,366.1 R15.1
N$28
  Top 0.254: R1012.2 LED1012.C
N$29
  Top 0.254: LED1016.C R1016.2
N$30
  Top 0.254: LED1017.C R1017.2
N$31
  Top 0.203: U20.6 107.64,365.85
  Top 0.254: 107.64,365.85 R14.1
N$32
  Top 0.254: LED1018.C R1018.2
N$73
  Top 0.254: U1.45 117.33,185.57 117.86,185.04 117.86,182.63 | 117.86,182.63 117.86,179.58 118.62,178.82 Y1.3 | C1.2 118.36,182.12 117.86,182.63
N$74
  Top 0.254: U1.44 116.83,184.56 R26.2
PPS  (via drill 0.6)
  Top 0.254: 167.26,239.9 193.55,213.61 206.5,213.61 207.8,212.32 J3.25 207.8,211.3 209.04,210.06 209.04,206.5 194.31,191.77 168.4,191.77 164.85,188.21 139.45,188.21 123.95,172.72 v123.95,172.34 | 167.26,239.9 149.22,257.94 146.43,257.94 146.05,258.32 146.05,261.11 139.19,267.97 139.19,272.8 | 139.19,272.8 139.19,273.81 | 139.19,273.81 139.19,329.18 | 139.19,329.18 139.19,340.87 143.26,344.93 v143.38,344.93 | v146.69,344.93 150.62,344.93 155.96,350.27 157.23,350.27 157.96,351.03 U9.3 | v123.95,170.05 124.33,169.67 124.33,161.8 v123.95,161.42 | v123.95,157.1 123.95,156.97 124.71,156.21 124.71,144.02 | 124.71,144.02 125.48,143.26 v127.89,143.26 | v130.68,143.26 v134.24,143.26 | v137.54,143.26 v142.62,143.26 | U11.3 150.11,143.26 v149.99,143.38 | 124.71,144.02 124.71,102.87 124.21,102.36 124.21,90.68 123.83,90.3 v123.7,90.3 | v123.7,88.01 v123.7,81.41 | v123.7,78.61 v123.7,68.96 | v123.7,63.88 123.7,62.74 | 123.7,62.74 129.54,56.9 v131.83,56.9 | v135.13,56.9 U13.3 | U12.3 109.47,48.51 123.7,62.74 | U10.3 111.76,239.52 v112.14,239.9 | v114.43,239.9 114.81,239.52 117.35,239.52 v117.73,239.9 | v120.02,239.9 120.4,239.52 124.71,239.52 v125.09,239.9 | v127.89,239.9 167.26,239.9 | U8.3 104.14,337.05 v104.52,337.44 | v109.35,337.44 109.73,337.06 111.76,337.06 v112.14,337.44 | v114.43,337.44 114.81,337.06 117.35,337.06 v117.73,337.44 | v120.02,337.44 120.4,337.06 131.32,337.06 139.19,329.18 | TP10.TESTPOINT 138.68,273.3 | 138.68,273.3 139.19,273.81 | 138.68,273.3 139.19,272.8
  Bottom 0.254: v143.38,344.93 v146.69,344.93 | v123.95,172.34 v123.95,170.05 | v123.95,161.42 v123.95,157.1 | v127.89,143.26 v130.68,143.26 | v134.24,143.26 v137.54,143.26 | v142.62,143.26 143,143.38 v149.99,143.38 | v123.7,90.3 v123.7,88.01 | v123.7,81.41 v123.7,78.61 | v123.7,68.96 v123.7,63.88 | v131.83,56.9 v135.13,56.9 | v112.14,239.9 v114.43,239.9 | v117.73,239.9 v120.02,239.9 | v125.09,239.9 v127.89,239.9 | v104.52,337.44 104.9,337.06 108.97,337.06 v109.35,337.44 | v112.14,337.44 112.52,337.06 114.05,337.06 v114.43,337.44 | v117.73,337.44 118.11,337.06 119.63,337.06 v120.02,337.44
SMBCLK  (via drill 0.6)
  Top 0.254: 202.18,188.72 215.19,201.73 215.19,267.16 214.2,268.15 J3.5 209.55,272.75 209.55,285.5 202.69,292.35 141.99,292.35 v141.55,292.79 | 202.18,188.72 197.61,184.15 171.7,184.15 168.15,180.59 142.75,180.59 136.14,173.99 v136.14,172.34 | v135.64,170.05 136.14,169.54 v136.14,159.89 | J4.5 52.65,171.27 53.85,172.47 55.63,172.47 56.39,171.7 56.39,163.58 59.44,160.53 91.95,160.53 93.02,161.59 v93.22,161.59 | v106.3,161.54 107.19,161.54 108.2,160.53 133.48,160.53 v133.86,160.91 | v136.14,156.97 136.14,155.96 | 136.14,155.96 136.14,90.81 v136.65,90.3 | U29.1 136.91,155.19 136.14,155.96 | v136.65,88.01 136.4,87.63 v136.4,81.41 | v136.4,77.22 136.4,75.95 137.16,75.18 U31.1 | U30.1 110.74,66.29 111.25,66.8 123.44,66.8 133.86,77.22 v134.49,77.22 | v97.28,161.59 97.48,161.59 98.55,160.53 102.11,160.53 103.12,161.54 v104.01,161.54 | v120.02,292.23 120.9,293.12 136.4,293.12 136.91,292.61 v137.08,292.61 136.72,292.24 R46.1 | v117.47,292.23 116.59,293.12 115.32,293.12 v114.43,292.23 | U28.1 108.46,290.83 108.84,291.21 | 108.84,291.21 109.86,292.23 v112.14,292.23 | U27.1 149.35,301.75 143,295.4 v143,293.88 | U26.1 98.04,295.91 101.6,292.35 107.06,292.35 v107.44,291.97 | v109.6,290.58 109.47,290.58 108.84,291.21 | 202.18,188.72 v202.18,187.45 | v203.45,186.18 205.49,184.15 210.82,184.15 TP2.TESTPOINT
  Bottom 0.254: v136.14,172.34 136.14,170.56 v135.64,170.05 | v136.14,156.97 v136.14,159.89 135.89,159.64 134.75,159.64 133.86,160.53 v133.86,160.91 | v136.65,90.3 v136.65,88.01 | v136.4,81.41 v136.4,77.22 v134.49,77.22 | v93.22,161.59 v97.28,161.59 | v106.3,161.54 v104.01,161.54 | v137.08,292.61 137.26,292.79 v141.55,292.79 141.91,292.79 v143,293.88 | v120.02,292.23 v117.47,292.23 | v114.43,292.23 v112.14,292.23 | v107.44,291.97 108.58,290.83 109.35,290.83 v109.6,290.58 | v202.18,187.45 v203.45,186.18
SMBDATA  (via drill 0.6)
  Top 0.254: 162.31,292.86 202.95,292.86 210.06,285.75 210.06,273.05 213.87,269.24 215.59,269.24 J3.3 216.69,267.23 215.65,266.19 215.65,201.42 203.2,188.98 203.2,187.2 | 162.31,292.86 145.03,292.86 | 145.03,292.86 144.02,292.86 | 144.02,292.86 142.85,292.86 v141.71,294 | 203.2,187.2 202.44,186.44 200.66,186.44 197.87,183.64 171.96,183.64 168.4,180.09 143,180.09 136.91,173.99 136.91,172.85 v137.41,172.34 | v136.91,170.05 136.65,169.8 136.65,160.66 v137.41,159.89 | v135.13,155.7 135.64,155.19 135.64,90.55 v135.38,90.3 | J4.3 55.09,171.17 53.85,169.93 53.85,164.85 58.67,160.02 92.1,160.02 92.89,160.81 93.52,160.81 93.62,160.71 v94.21,160.71 | v106.93,160.53 107.44,160.53 107.95,160.02 134.24,160.02 134.75,160.53 v134.75,161.8 | U29.2 137.41,153.92 v137.03,154.31 | v135.38,88.01 135.38,87.88 135.89,87.38 135.89,82.55 v135.38,82.04 | U31.2 137.16,73.91 135.38,75.69 v135.38,78.49 134.37,78.49 123.19,67.31 111.25,67.31 111,67.56 U30.2 | v96.29,160.71 96.9,160.71 97,160.81 97.59,160.81 98.4,160 102.84,160 v103.38,160.53 | v137.39,293.75 137.29,293.75 137.16,293.62 120.14,293.62 v120.02,293.5 | v117.47,293.5 117.35,293.62 114.55,293.62 v114.43,293.5 | U28.2 107.19,281.69 107.95,282.45 107.95,291.08 109.73,292.86 | v112.14,293.5 110.36,293.5 109.73,292.86 | U27.2 150.62,304.55 162.31,292.86 | U26.2 99.31,295.4 101.85,292.86 109.73,292.86 | R45.1 144.53,293.37 | 144.53,293.37 144.02,292.86 | 144.53,293.37 145.03,292.86 | TP1.TESTPOINT 205.74,185.42 203.96,187.2 203.2,187.2
  Bottom 0.254: v137.41,172.34 136.91,171.83 v136.91,170.05 | 137.03,156.59 137.03,159.51 v137.41,159.89 136.53,160.78 135.25,160.78 134.75,161.29 v134.75,161.8 | 137.03,156.59 136.14,155.7 v135.13,155.7 | v103.38,160.53 v106.93,160.53 | 137.03,156.59 v137.03,154.31 | v135.38,90.3 v135.38,88.01 | v135.38,82.04 v135.38,78.49 | v94.21,160.71 v96.29,160.71 | v141.71,294 141.71,293.98 141.48,293.75 v137.39,293.75 | v120.02,293.5 119.89,293.62 117.6,293.62 v117.47,293.5 | v114.43,293.5 114.3,293.62 112.27,293.62 v112.14,293.5
USB_SUSPEND_STATUS
  Top 0.254: U1.1 120.86,187.75 122.17,186.44 125.48,186.44 126.75,187.71 128.27,187.71 129.54,186.44 TP31.TESTPOINT
VBATT+
  Top 0.508: J4.17 37.31,171.17 36.07,169.93 36.07,167.39 36.58,166.88
  Top 1.27: J9.1 50.29,143.51 36.58,157.23 36.58,166.88
  Bottom 0.508: J4.17 37.31,182.09 38.35,183.13 38.35,186.44 TP14.TESTPOINT
VBATT-
  Top 1.27: J9.2 54.28,142.06 38.61,157.73 38.61,167.44 J4.18
  Bottom 0.508: J4.18 37.41,168.73 38.61,169.93 38.61,181.1 40.39,182.88 TP15.TESTPOINT
VCC_BACKPLANE  (via drill 0.6, 1.2)
  Top 0.203: U20.9 105.92,361.7 105.52,362.09 | U21.9 127.4,362.2 C65.2 | U25.9 150.62,89.15
  Top 0.254: C64.2 105.52,362.09 | C16.1 149.46,324.22 149.35,324.1 U27.18 | U23.9 157.59,174.75 C67.2 | U1.46 117.83,185.7 118.11,185.42 118.33,185.64 U1.47 118.33,187.42 118.62,187.71 118.62,188.47 117.73,189.36 117.73,190.37 118.61,191.25 U1.8 121.15,191.25 121.16,191.26 | U1.9 121.14,191.75 121.16,191.77 | C69.2 150.62,89.15 | S12.5 147.43,67.82 C75.1 | S11.5 46.37,96.01 C74.1 | U24.9 93.23,88.52 C68.2 93.09,88.39 v91.82,89.66 | U22.9 91.96,228.73 C66.2 | U3.1 159,339.34 158.64,339.71 C23.1 | U19.1 152.3,64.76 C61.1 152.16,65.52 151.89,65.79
  Bottom 0.203: v87.12,227.08 v88.39,228.35 | v88.65,229.74 v87.5,230.89
  Bottom 0.254: v104.39,365.89 v104.39,364.11 | v89.41,362.97 v89.41,360.43 | v135.13,365.89 v135.13,363.6 | v164.34,365.89 v164.34,363.6 | v129.48,359.47 v128.22,360.73 | v130.3,364.11 v130.3,365.89 | v143.89,355.85 v146.69,355.85 | v157.48,355.85 155.7,355.85 v155.19,355.35 | v146.69,346.96 v143.38,346.96 | v131.42,334.22 v133.4,336.19 | v138.3,338.07 v140.08,338.07 | v143.38,342.14 v146.69,342.14 | v144.65,336.93 v147.07,339.34 | v150.62,342.9 v152.65,342.9 v153.92,341.63 | v137.29,324.36 v141.1,324.36 | v137.29,316.99 v141.1,316.99 | v138.68,157.1 v138.68,159.89 | v142.88,161.8 v141.73,160.66 | v143.13,163.96 v143.13,165.74 | v160.15,167.26 v161.42,168.53 | v159.51,173.35 v160.66,172.21 | v160.4,175.26 v161.54,176.4 | v181.1,192.66 v181.1,190.37 | v152.15,185.55 v152.15,183.26 | v202.95,191.39 v204.85,189.48 | v137.92,177.67 v139.83,175.77 | v128.45,178.56 v130.07,176.95 | v156.08,153.67 v154.69,155.07 | v151.89,92.08 v151.89,90.35 | v153.42,87.96 v153.42,86.23 | v125.6,59.69 v126.75,60.83 | v137.16,51.69 v138.68,53.21 | v130.43,61.34 v132.72,61.34 | v140.97,57.78 v140.97,56.01 | v137.54,163.58 v134.75,163.58 | v130.68,163.58 v128.4,163.58 | v125.73,163.58 v123.44,163.58 | v132.72,164.21 v132.72,166.5 | v130.68,167.39 v128.4,167.39 | v115.57,172.34 v115.57,170.05 | v106.35,115.83 v104.07,115.83 | v106.35,144.53 v104.07,144.53 | v93.4,168.91 v95.56,168.91 | v98.61,174.75 v96.45,174.75 | v99.5,181.36 v101.66,181.36 | v95.66,191.04 v97.21,189.49 | v89.15,87.12 v90.68,88.65 | v91.82,92.08 v91.82,89.66 | v120.27,60.45 v121.41,59.31 | v110.62,50.8 v111.76,49.66 | v105.54,54.86 v107.82,54.86 | v107.82,59.18 v105.54,59.18 | v113.16,61.72 v113.16,64.26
